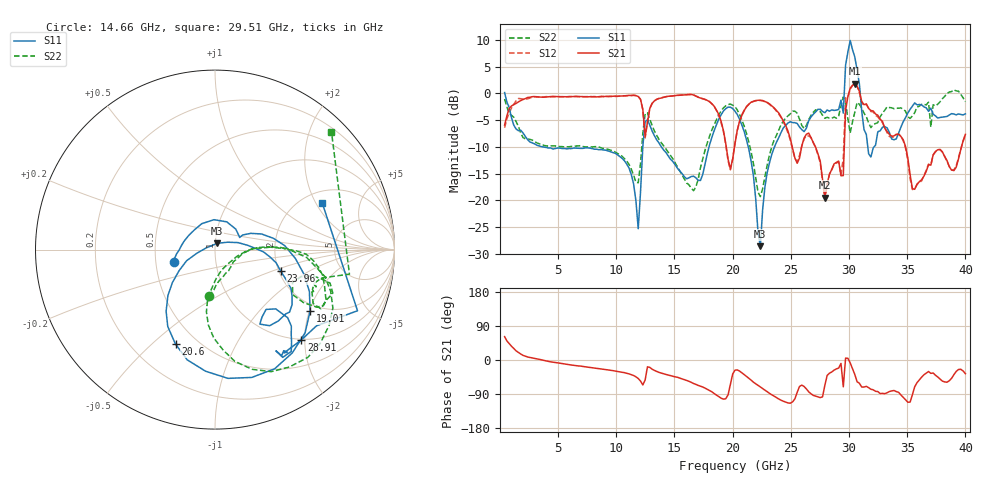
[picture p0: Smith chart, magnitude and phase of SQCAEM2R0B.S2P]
! Network Analyzer HP8722ES.07.66: Jul 25, 2000 Serial No. US39175408
! 26 Oct 2004  11:39:55
! Frequency  S11  S21  S12  S22
# HZ  S  DB R  50
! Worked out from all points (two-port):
!   201 points, 400 MHz to 40 GHz, reference 50 ohm
!   highest |S21| = 1.77 dB at 30.5 GHz (marker M1); lowest = -19.5 dB at 27.92 GHz (marker M2)
!   |S21| within 3 dB of the highest: 1.917 GHz to 12.09 GHz (10.17 GHz wide, 145 % of centre); 13.41 GHz to 17.72 GHz (4.309 GHz wide, 27.7 % of centre)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
!   lowest |S11| = -28.6 dB at 22.38 GHz (marker M3), VSWR 1.08, Z = 51.1 + j3.6 ohm
!   |S11| at or under -10 dB: 3.641 GHz to 12.28 GHz (8.636 GHz wide, 109 % of centre); 13.87 GHz to 17.97 GHz (4.102 GHz wide, 25.8 % of centre); 21.34 GHz to 23.6 GHz (2.26 GHz wide, 10.1 % of centre)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
!   |S22| runs from -19.3 to 0.7 dB; largest |S21 - S12| = 0.22
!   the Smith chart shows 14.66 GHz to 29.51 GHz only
!   S11 on the Smith chart (normalised r, x): 14.66 GHz: 0.62, -0.09; 19.01 GHz: 1.78, -2.03; 20.6 GHz: 0.38, -0.60; 23.96 GHz: 2.05, -0.58; 28.91 GHz: 0.98, -1.92; 29.51 GHz: 2.51, +2.26
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4e8  0.14 -29.4  -5.93 61.5  -6.44 67.2  -1.06 -21.2
7.132e9  -10.29 -112.6  -0.61 -17.1  -0.66 -17.9  -9.94 -103.9
1.1884e10  -25.31 127.0  -0.60 -48.9  -0.59 -49.6  -16.71 -52.8
1.2478e10  -5.30 -48.7  -8.04 -52.8  -8.34 -51.6  -3.78 -50.9
1.3666e10  -9.28 -139.4  -0.97 -32.7  -0.96 -33.2  -8.63 -100.4
1.4656e10  -12.33 -162.8  -0.54 -41.1  -0.53 -42.0  -11.61 -97.6
1.9012e10  -4.00 -32.9  -5.28 -100.8  -5.52 -102.1  -3.29 -19.8
2.02e10  -3.36 -94.4  -9.40 -26.8  -9.25 -27.3  -2.51 -65.2
2.0596e10  -4.87 -112.7  -5.20 -29.3  -5.24 -30.2  -3.98 -79.9
2.2378e10  -28.57 70.3  -1.30 -71.0  -1.33 -72.2  -19.30 -42.4
2.3962e10  -8.28 -18.2  -3.67 -102.9  -3.88 -104.1  -6.85 -0.9
2.6932e10  -3.90 -48.3  -9.24 -93.4  -9.22 -94.9  -3.51 -16.2
2.7922e10  -3.63 -59.0  -19.48 -66.7  -19.74 -65.5  -4.66 -22.8
2.8912e10  -3.14 -46.4  -12.91 -23.5  -13.02 -24.1  -4.65 -18.5
2.9506e10  -3.72 23.5  -15.37 -70.8  -12.12 -59.8  -0.70 45.3
2.9704e10  5.26 -42.5  -3.15 5.1  -0.83 8.0  -1.62 -91.3
3.01e10  9.88 -77.5  0.95 -7.7  0.77 -9.3  -7.42 -29.0
3.0496e10  6.79 -102.7  1.77 -38.3  1.78 -38.7  -3.55 -27.7
3.0694e10  4.33 51.2  1.29 -57.4  1.36 -57.5  -1.73 145.5
3.1486e10  -7.70 -117.0  -1.97 -69.5  -2.10 -71.9  -4.35 -44.9
3.3466e10  -7.32 -59.5  -7.67 -83.2  -8.05 -83.5  -2.66 -20.1
4e10  -3.84 -69.4  -7.68 -36.1  -7.70 -36.3  -1.55 -12.3
